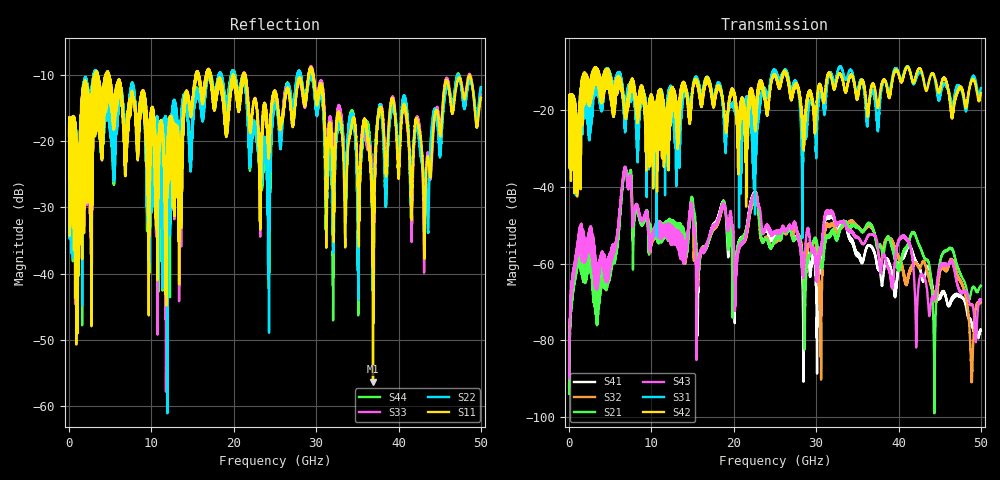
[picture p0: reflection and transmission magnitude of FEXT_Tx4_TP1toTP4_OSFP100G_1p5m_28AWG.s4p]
! Touchstone data
! Created: 27-Feb-2019 by IdEM 12 (12.1.0)
! COMMENTS
!  Created Wed Feb 27 09:43:39 2019
!  64 Port Network Data from SP1.SP block
!  freq  magS1_1  angS1_1  magS1_2  angS1_2  magS1_3  angS1_3  magS1_4  angS1_4
!  magS1_5  angS1_5  magS1_6  angS1_6  magS1_7  angS1_7  magS1_8  angS1_8
!  magS1_9  angS1_9  magS1_10  angS1_10  magS1_11  angS1_11  magS1_12  angS1_12
!  magS1_13  angS1_13  magS1_14  angS1_14  magS1_15  angS1_15  magS1_16  angS1_16
!  magS1_17  angS1_17  magS1_18  angS1_18  magS1_19  angS1_19  magS1_20  angS1_20
!  magS1_21  angS1_21  magS1_22  angS1_22  magS1_23  angS1_23  magS1_24  angS1_24
!  magS1_25  angS1_25  magS1_26  angS1_26  magS1_27  angS1_27  magS1_28  angS1_28
!  magS1_29  angS1_29  magS1_30  angS1_30  magS1_31  angS1_31  magS1_32  angS1_32
!  magS1_33  angS1_33  magS1_34  angS1_34  magS1_35  angS1_35  magS1_36  angS1_36
!  magS1_37  angS1_37  magS1_38  angS1_38  magS1_39  angS1_39  magS1_40  angS1_40
!  magS1_41  angS1_41  magS1_42  angS1_42  magS1_43  angS1_43  magS1_44  angS1_44
!  magS1_45  angS1_45  magS1_46  angS1_46  magS1_47  angS1_47  magS1_48  angS1_48
!  magS1_49  angS1_49  magS1_50  angS1_50  magS1_51  angS1_51  magS1_52  angS1_52
!  magS1_53  angS1_53  magS1_54  angS1_54  magS1_55  angS1_55  magS1_56  angS1_56
!  magS1_57  angS1_57  magS1_58  angS1_58  magS1_59  angS1_59  magS1_60  angS1_60
!  magS1_61  angS1_61  magS1_62  angS1_62  magS1_63  angS1_63  magS1_64  angS1_64
!  magS2_1  angS2_1  magS2_2  angS2_2  magS2_3  angS2_3  magS2_4  angS2_4
!  magS2_5  angS2_5  magS2_6  angS2_6  magS2_7  angS2_7  magS2_8  angS2_8
!  magS2_9  angS2_9  magS2_10  angS2_10  magS2_11  angS2_11  magS2_12  angS2_12
!  magS2_13  angS2_13  magS2_14  angS2_14  magS2_15  angS2_15  magS2_16  angS2_16
!  magS2_17  angS2_17  magS2_18  angS2_18  magS2_19  angS2_19  magS2_20  angS2_20
!  magS2_21  angS2_21  magS2_22  angS2_22  magS2_23  angS2_23  magS2_24  angS2_24
!  magS2_25  angS2_25  magS2_26  angS2_26  magS2_27  angS2_27  magS2_28  angS2_28
!  magS2_29  angS2_29  magS2_30  angS2_30  magS2_31  angS2_31  magS2_32  angS2_32
!  magS2_33  angS2_33  magS2_34  angS2_34  magS2_35  angS2_35  magS2_36  angS2_36
!  magS2_37  angS2_37  magS2_38  angS2_38  magS2_39  angS2_39  magS2_40  angS2_40
!  magS2_41  angS2_41  magS2_42  angS2_42  magS2_43  angS2_43  magS2_44  angS2_44
!  magS2_45  angS2_45  magS2_46  angS2_46  magS2_47  angS2_47  magS2_48  angS2_48
!  magS2_49  angS2_49  magS2_50  angS2_50  magS2_51  angS2_51  magS2_52  angS2_52
!  magS2_53  angS2_53  magS2_54  angS2_54  magS2_55  angS2_55  magS2_56  angS2_56
!  magS2_57  angS2_57  magS2_58  angS2_58  magS2_59  angS2_59  magS2_60  angS2_60
!  magS2_61  angS2_61  magS2_62  angS2_62  magS2_63  angS2_63  magS2_64  angS2_64
!  magS3_1  angS3_1  magS3_2  angS3_2  magS3_3  angS3_3  magS3_4  angS3_4
!  magS3_5  angS3_5  magS3_6  angS3_6  magS3_7  angS3_7  magS3_8  angS3_8
!  magS3_9  angS3_9  magS3_10  angS3_10  magS3_11  angS3_11  magS3_12  angS3_12
!  magS3_13  angS3_13  magS3_14  angS3_14  magS3_15  angS3_15  magS3_16  angS3_16
!  magS3_17  angS3_17  magS3_18  angS3_18  magS3_19  angS3_19  magS3_20  angS3_20
!  magS3_21  angS3_21  magS3_22  angS3_22  magS3_23  angS3_23  magS3_24  angS3_24
!  magS3_25  angS3_25  magS3_26  angS3_26  magS3_27  angS3_27  magS3_28  angS3_28
!  magS3_29  angS3_29  magS3_30  angS3_30  magS3_31  angS3_31  magS3_32  angS3_32
!  magS3_33  angS3_33  magS3_34  angS3_34  magS3_35  angS3_35  magS3_36  angS3_36
!  magS3_37  angS3_37  magS3_38  angS3_38  magS3_39  angS3_39  magS3_40  angS3_40
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# Hz S MA R 50
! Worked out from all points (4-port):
!   5000 points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, 10 MHz to 50 GHz, reference 50 ohm
!   strongest paths, dB at 10 MHz, 12.51 GHz, 25.01 GHz, 37.51 GHz, 50 GHz:
!     S42: -19.6, -19.1, -10.7, -19.1, -15.4
!     S31: -19.6, -16.6, -9.8, -25.4, -14.2
!     S43: -89.8, -51.5, -51.6, -55.7, -69.3
!     S21: -94.0, -49.3, -53.7, -55.9, -65.7
!     S32: -91.6, -50.5, -54.3, -56.9, -70.0
!     S41: -92.1, -50.3, -52.5, -61.3, -77.4
!   lowest |S11| = -56.3 dB at 36.9 GHz (marker M1), VSWR 1.00, Z = 50.1 + j0.121 ohm
!   |S11| at or under -10 dB: 4.861 GHz to 15.4 GHz (10.54 GHz wide, 104 % of centre); 21.38 GHz to 29.07 GHz (7.682 GHz wide, 30.5 % of centre); 29.66 GHz to end of sweep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
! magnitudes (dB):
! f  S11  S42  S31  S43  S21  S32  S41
! 10 MHz  -19.1  -19.6  -19.6  -89.8  -94.0  -91.6  -92.1
! 6.83 GHz  -20.4  -20.8  -19.6  -35.0  -35.1  -34.9  -35.0
! 15.61 GHz  -9.4  -12.8  -12.1  -62.5  -63.2  -66.5  -78.2
! 22.56 GHz  -13.6  -23.1  -28.5  -41.5  -41.9  -42.6  -41.3
! 30.51 GHz  -11.2  -13.2  -15.8  -57.9  -60.6  -70.2  -62.3
! 36.9 GHz  -56.3  -12.9  -14.9  -52.5  -50.9  -51.2  -56.2
! 50 GHz  -13.4  -15.4  -14.2  -69.3  -65.7  -70.0  -77.4
